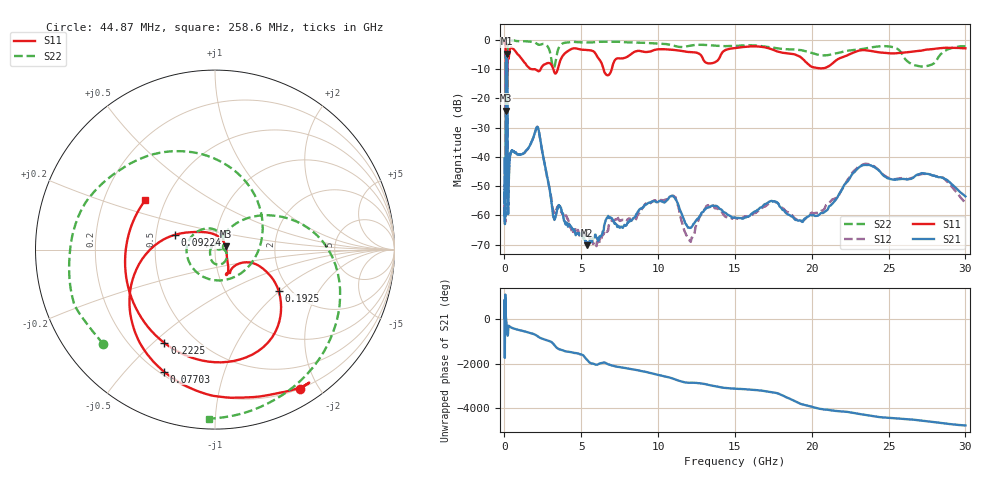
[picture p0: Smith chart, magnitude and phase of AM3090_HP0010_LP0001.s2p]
! Date/Time: Thu, Feb 28, 2019 1:55 PM
! Network Analyzer: Agilent Technologies E8364B Rev: A.07.50.67
! Sweep from 0.010 to 30.000 GHz, 1601 Points, Sweep Type: LOG
! Power Supply: 5.023 V, 0.002 A
# Hz S DB R 50
!freq MagS11 AngS11 MagS21 AngS21 MagS12 AngS12 MagS22 AngS22
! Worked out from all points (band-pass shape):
!   1601 points, 10 MHz to 30 GHz, reference 50 ohm
!   highest |S21| = -4.71 dB at 136.3 MHz (marker M1); lowest = -70.3 dB at 5.392 GHz (marker M2)
!   |S21| within 3 dB of the highest: 100 MHz to 177.7 MHz (77.64 MHz wide, 55.9 % of centre)
!   lowest |S11| = -24.1 dB at 99.43 MHz (marker M3), VSWR 1.13, Z = 56.2 + j2.16 ohm
!   |S11| at or under -10 dB: 1.995 GHz to 2.355 GHz (360.6 MHz wide, 16.6 % of centre); 3.181 GHz to 3.465 GHz (283.8 MHz wide, 8.54 % of centre); 6.451 GHz to 6.979 GHz (527.7 MHz wide, 7.86 % of centre)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
!   |S22| runs from -36.5 to -0.1 dB; largest |S21 - S12| = 0.013
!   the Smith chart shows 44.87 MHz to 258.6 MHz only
!   S11 on the Smith chart (normalised r, x): 44.87 MHz: 0.20, -1.76; 77.03 MHz: 0.22, -0.64; 92.24 MHz: 0.63, +0.11; 192.5 MHz: 1.75, -0.98; 222.5 MHz: 0.34, -0.54; 258.6 MHz: 0.39, +0.28
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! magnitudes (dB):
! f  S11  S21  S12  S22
! 10 MHz  -0.3  -40.5  -42.4  -0.6
! 38.04 MHz  -0.5  -59.0  -59.8  -1.4
! 44.87 MHz  -0.8  -53.7  -58.1  -1.8
! 77.03 MHz  -2.7  -44.9  -44.0  -5.2
! 92.24 MHz  -12.4  -13.9  -13.9  -15.5
! 99.43 MHz  -24.1  -8.0  -7.9  -16.5
! 127.1 MHz  -16.5  -4.8  -4.8  -36.3
! 136.3 MHz  -16.5  -4.7  -4.7  -28.6
! 144.7 MHz  -16.2  -4.8  -4.8  -22.2
! 170.7 MHz  -15.7  -6.4  -6.4  -33.2
! 192.5 MHz  -7.5  -17.6  -17.6  -10.4
! 222.5 MHz  -4.6  -56.6  -57.9  -1.4
! 258.6 MHz  -6.4  -52.8  -54.6  -0.5
! 550.5 MHz  -3.0  -38.1  -38.0  -0.2
! 2.084 GHz  -10.3  -30.1  -30.0  -1.2
! 3.22 GHz  -10.7  -60.7  -58.7  -9.6
! 5.392 GHz  -3.4  -70.3  -66.0  -0.8
! 7.926 GHz  -5.9  -63.5  -61.5  -0.8
! 10.76 GHz  -3.3  -53.6  -53.6  -1.6
! 19.61 GHz  -7.5  -61.0  -61.0  -3.8
! 23.48 GHz  -3.5  -42.7  -42.3  -2.9
! 30 GHz  -2.8  -53.5  -55.7  -2.1
